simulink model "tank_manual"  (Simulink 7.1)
settings: Solver=ode45  StartTime=0.0  StopTime=Inf  RelTol=1e-3
libraries: simulink x2

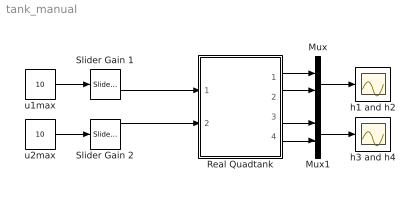
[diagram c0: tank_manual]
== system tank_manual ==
  Mux : Mux  Inputs=2
  Mux1 : Mux  Inputs=2
  Real Quadtank : Subsystem  AncestorBlock=tank/Real Quadtank  mask{h=0.05}
  Slider Gain 1 : simulink/Math Operations/Slider Gain  SystemSampleTime=-1  low=0  gain=0  high=1
  Slider Gain 2 : simulink/Math Operations/Slider Gain  SystemSampleTime=-1  low=0  gain=0  high=1
  h1 and h2 : Scope
  h3 and h4 : Scope
  u1max : Constant  Value=10  OutDataType=sfix(16)  OutScaling=2^0
  u2max : Constant  Value=10  OutDataType=sfix(16)  OutScaling=2^0
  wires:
  Real Quadtank/1(y1) -> Mux/1
  Real Quadtank/2(y2) -> Mux/2
  Real Quadtank/3(y3) -> Mux1/1
  Real Quadtank/4(y4) -> Mux1/2
  Mux1/1 -> h3 and h4/1
  Mux/1 -> h1 and h2/1
  u1max/1 -> Slider Gain 1/1
  Slider Gain 1/1 -> Real Quadtank/1(u1)
  u2max/1 -> Slider Gain 2/1
  Slider Gain 2/1 -> Real Quadtank/2(u2)

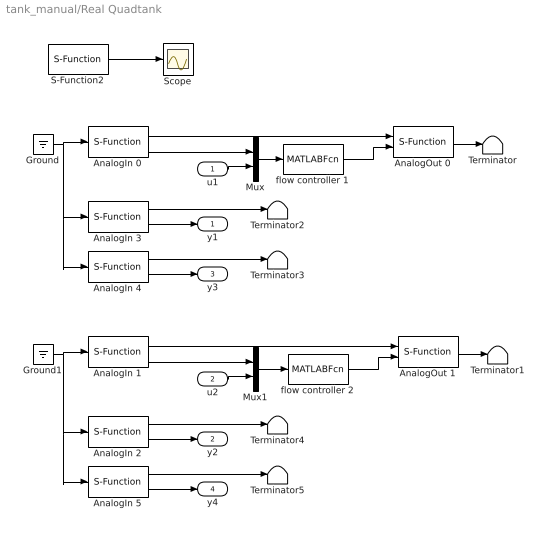
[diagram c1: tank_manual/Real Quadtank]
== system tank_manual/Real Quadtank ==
  u1 : Inport  OutDataType=sfix(16)  OutScaling=2^0
  u2 : Inport  Port=2  OutDataType=sfix(16)  OutScaling=2^0
  AnalogIn 0 : S-Function  FunctionName=analogin  Parameters=h [35]  EnableBusSupport=off
  AnalogIn 1 : S-Function  FunctionName=analogin  Parameters=h [34]  EnableBusSupport=off
  AnalogIn 2 : S-Function  FunctionName=analogin  Parameters=h [33]  EnableBusSupport=off
  AnalogIn 3 : S-Function  FunctionName=analogin  Parameters=h [31]  EnableBusSupport=off
  AnalogIn 4 : S-Function  FunctionName=analogin  Parameters=h [30]  EnableBusSupport=off
  AnalogIn 5 : S-Function  FunctionName=analogin  Parameters=h [32]  EnableBusSupport=off
  AnalogOut 0 : S-Function  FunctionName=analogout  Parameters=h [31]  EnableBusSupport=off
  AnalogOut 1 : S-Function  FunctionName=analogout  Parameters=h [30]  EnableBusSupport=off
  Ground : Ground
  Ground1 : Ground
  Mux : Mux  Inputs=2
  Mux1 : Mux  Inputs=2
  S-Function2 : S-Function  FunctionName=realtimer  Parameters=h  EnableBusSupport=off
  Scope : Scope
  Terminator{,1..5} (6 alike) : Terminator
  flow controller 1 : MATLABFcn  MATLABFcn=flowCtrl1  SampleTime=0.01
  flow controller 2 : MATLABFcn  MATLABFcn=flowCtrl2  SampleTime=0.01
  y1 : Outport  OutDataType=sfix(16)  OutScaling=2^0
  y2 : Outport  Port=2  OutDataType=sfix(16)  OutScaling=2^0
  y3 : Outport  Port=3  OutDataType=sfix(16)  OutScaling=2^0
  y4 : Outport  Port=4  OutDataType=sfix(16)  OutScaling=2^0
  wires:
  S-Function2/1 -> Scope/1
  AnalogIn 0/1 -> AnalogOut 0/1
  AnalogOut 0/1 -> Terminator/1
  AnalogIn 1/1 -> AnalogOut 1/1
  AnalogOut 1/1 -> Terminator1/1
  AnalogIn 3/2 -> y1/1
  AnalogIn 4/2 -> y3/1
  Ground/1 -> AnalogIn 0/1, AnalogIn 3/1, AnalogIn 4/1
  AnalogIn 3/1 -> Terminator2/1
  AnalogIn 4/1 -> Terminator3/1
  AnalogIn 2/2 -> y2/1
  AnalogIn 5/2 -> y4/1
  Ground1/1 -> AnalogIn 5/1, AnalogIn 2/1, AnalogIn 1/1
  AnalogIn 2/1 -> Terminator4/1
  AnalogIn 5/1 -> Terminator5/1
  u1/1 -> Mux/2
  Mux/1 -> flow controller 1/1
  flow controller 1/1 -> AnalogOut 0/2
  u2/1 -> Mux1/2
  Mux1/1 -> flow controller 2/1
  flow controller 2/1 -> AnalogOut 1/2
  AnalogIn 1/2 -> Mux1/1
  AnalogIn 0/2 -> Mux/1
